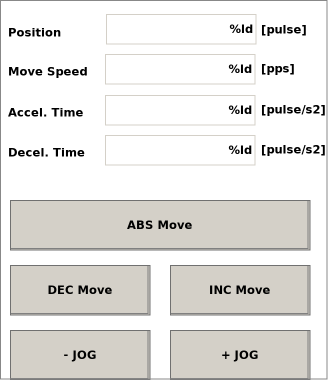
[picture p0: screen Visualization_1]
VISUALIZATION Visualization_1  // 328x380
    Label (5,20 80x25), "Position"
    Label (258,17 50x25), "[pulse]"
    Textfield (105,54 150x30), "%ld", text variable: main.profile_velocity
        OnMouseClick: write the text variable via Default, min 1, max 2500000, format 10000
    Label (5,59 80x25), "Move Speed"
    Label (258,56 50x25), "[pps]"
    Textfield (105,95 150x30), "%ld", text variable: main.profile_acceleration
        OnMouseClick: write the text variable via Default, min 1000, max 1000000000, format 1000000
    Label (5,100 81x25), "Accel. Time"
    Label (258,97 70x25), "[pulse/s2]"
    Textfield (105,135 150x30), "%ld", text variable: main.profile_deceleration
        OnMouseClick: write the text variable via Default, min 1000, max 1000000000, format 1000000
    Label (5,140 81x25), "Decel. Time"
    Label (258,137 69x25), "[pulse/s2]"
    Button (10,330 140x50), "- JOG"
        tap move_prg.minus_jog
    Button (170,330 140x50), "+ JOG"
        tap move_prg.plus_jog
    Button (10,265 140x50), "DEC Move"
        tap move_prg.dec_move
    Button (170,265 140x50), "INC Move"
        tap move_prg.inc_move
    Button (10,200 300x50), "ABS Move"
        tap move_prg.abs_move
    Textfield (106,14 150x30), "%ld", text variable: move_prg.target_pos_g
        OnMouseClick: write the text variable via Default, min -2147483648, max 2147483647, format 10000
END_VISUALIZATION
